FUNCTION_BLOCK FB_SboControl EXTENDS FB_AsyncServiceResultClass IMPLEMENTS I_AcsiDataAccessEventClass, I_AcsiDataAccessCompletionClass
VAR
	(* Interface pointer to controllable DO *)
	_ipCtrl					: I_AcsiCommonControllableDataClass;
	(* CDC type of the controllable DO *)
	_eType					: E_AcsiCDCType;
	(* Interface pointer to value of 'Beh' DO of parent LN *)
	_ipBehVal				: I_AcsiDATypeBeh;
	(* Interface pointer to DO containing stepsize information for BAC *)
	_ipStepSize				: I_AcsiDATypeAnalogueValue;
	
	(* State of control state machine *)
	_eControlState			: E_SboControlState;
	(* Interface pointer to association for the current control procedure *)
	_ipCurrentAA			: I_ScsmAssociationClass;
	(* IP address of the client for the current control procedure *)
	_stCurrrentIp			: ST_SockAddr;
	(* Timer to monitor 'sboTimeout' *)
	_fbSboTimer				: TON;
	
	(* Interface pointer to LastApplError request service *)
	_ipLastApplErrorReq		: I_AsyncServiceResultClass;
	(* State of LastApplError transmission *)
	_nLastApplErrorReqState	: BYTE;
	(* Interface pointer to CommandTermination request service *)
	_ipCmdTermReq			: I_AsyncServiceResultClass;
	(* State of CommandTermination transmission *)
	_nCmdTermReqState		: BYTE;
	
	(* Indicates whether this function block has been initialized *)
	bInit					: BOOL;
	(* Indicates whether the ControlState changed in the last cycle *)
	bNewState				: BOOL;
	(* Indicates whether a valid Oper_req was received *)
	bOperReq				: BOOL;
	(* Indicates whether a valid SelVal_req was received *)
	bSelValReq					: BOOL;
	(* Indicates whether a valid Cancel_req was received *)
	bCancelReq				: BOOL;
	(* Token for CompletionWaitEvent *)
	fbCompletion			: FB_AcsiServiceResultClass;
	(* Token for CompletionWaitEvent of SelVal_req *)
	fbSelValCompletion		: FB_AcsiServiceResultClass;
	(* Token for CompletionWaitEvent of Oper_req *)
	fbOperCompletion		: FB_AcsiServiceResultClass;
	(* Token for CompletionWaitEvent of Cancel_req *)
	fbCancelCompletion		: FB_AcsiServiceResultClass;
END_VAR

(*
	This method is called when Cancel_req is received.
	It shall check whether the Cancel request is valid and return FALSE as well as an error code if it is not.
*)
METHOD PROTECTED _CheckCancelReq : BOOL
VAR_INPUT
	(* Additional data access info *)
	ipDai			: I_AcsiDataAccessInfoClass;
END_VAR
VAR_OUTPUT
	(* Error code for negative response *)
	eError			: E_AcsiServiceError;
END_VAR
VAR
	(* Interface pointer to application association *)
	ipAA			: I_ScsmAssociationClass;
	(* Address of the client that sent the Cancel_req *)
	stRemoteAddr	: ST_SockAddr;
END_VAR
IF (_ipCtrl <> 0) AND_THEN (_ipCtrl.ipCancel <> 0) THEN
	ScsmAssociation_From_Dai(in:=ipDai, out=>ipAA);
	(* Don't allow control if 'ctlModel' is set to 'status-only' *)
	IF (_ipCtrl.ipCtlModel <> 0) AND_THEN (_ipCtrl.ipCtlModel.eValue = E_AcsiCtlModels.StatusOnly) THEN
		_SendLastApplError(ipAA:=ipAA,
			ipCtrlData:=_ipCtrl.ipCancel,
			eError:=E_AcsiApplError.NoError,
			ipOrigin:=_ipCtrl.ipCancel.ipOrigin,
			ipCtlNum:=_ipCtrl.ipCancel.ipCtlNum,
			eAddCause:=E_AcsiApplAddCause.Unknown);
		RETURN;
	
	(* Cancel is always allowed in state 'Unselected' *)
	ELSIF (_eControlState = E_SboControlState.Unselected) THEN
		_CheckCancelReq:=TRUE;
		RETURN;
	
	(* Cancel is only allowed by the same client that sent the last accepted SelVal_req *)
	ELSIF (RemoteAddress_From_ScsmAssociation(in:=ipAA, out=>stRemoteAddr)) AND_THEN (stRemoteAddr.sAddr <> _stCurrrentIp.sAddr) THEN
		_SendLastApplError(ipAA:=ipAA,
			ipCtrlData:=_ipCtrl.ipCancel,
			eError:=E_AcsiApplError.NoError,
			ipOrigin:=_ipCtrl.ipCancel.ipOrigin,
			ipCtlNum:=_ipCtrl.ipCancel.ipCtlNum,
			eAddCause:=E_AcsiApplAddCause.LockedByOtherClient);
		RETURN;
	
	(* Cancel is not allowed in state 'WaitForChange' *)
	ELSIF (_eControlState = E_SboControlState.WaitForChange) THEN
		_SendLastApplError(ipAA:=ipAA,
			ipCtrlData:=_ipCtrl.ipCancel,
			eError:=E_AcsiApplError.NoError,
			ipOrigin:=_ipCtrl.ipCancel.ipOrigin,
			ipCtlNum:=_ipCtrl.ipCancel.ipCtlNum,
			eAddCause:=E_AcsiApplAddCause.CommandAlreadyInExecution);
		RETURN;
	
	(* Cancel is valid *)
	ELSE
		_CheckCancelReq:=TRUE;
	END_IF
END_IF
END_METHOD

(*
	Checks if the value of 'ctlVal' is valid.
	Return value: TRUE => success, FALSE => failure
*)
METHOD PROTECTED _CheckCtlVal : BOOL
VAR_INPUT
	(* Value of 'ctlVal' DA *)
	uCtlVal			: U_AcsiCtlVal;
END_VAR
VAR_OUTPUT
	(* Error *)
	eError			: E_AcsiApplError;
	(* Application error code *)
	eAddCause		: E_AcsiApplAddCause;
END_VAR
IF (_ipCtrl = 0) OR_ELSE (_eType = E_AcsiCDCType.none) THEN
	RETURN;
END_IF

CASE _eType OF
	E_AcsiCDCType.SPC:
		IF (_ipCtrl.ipStVal_BOOLEAN = 0) THEN
			RETURN;
		END_IF
		IF (uCtlVal.SPC = _ipCtrl.ipStVal_BOOLEAN.bValue) THEN
			eError:=E_AcsiApplError.NoError;
			eAddCause:=E_AcsiApplAddCause.PositionReached;
		ELSE
			_CheckCtlVal:=TRUE;
		END_IF
	
	E_AcsiCDCType.DPC:
		IF (_ipCtrl.ipStVal_Dbpos = 0) THEN
			RETURN;
		END_IF
		IF ((SEL(uCtlVal.DPC, E_AcsiDbpos.Off, E_AcsiDbpos.On)) = _ipCtrl.ipStVal_Dbpos.eValue) THEN
			eError:=E_AcsiApplError.NoError;
			eAddCause:=E_AcsiApplAddCause.PositionReached;
		ELSE
			_CheckCtlVal:=TRUE;
		END_IF
	
	E_AcsiCDCType.INC:
		IF (_ipCtrl.ipStVal_INT32 = 0) THEN
			RETURN;
		END_IF
		IF (uCtlVal.INC = _ipCtrl.ipStVal_INT32.iValue) THEN
			eError:=E_AcsiApplError.NoError;
			eAddCause:=E_AcsiApplAddCause.PositionReached;
		ELSE
			_CheckCtlVal:=TRUE;
		END_IF
		
	E_AcsiCDCType.ENC:
		IF (_ipCtrl.ipStVal_ENUMERATED = 0) THEN
			RETURN;
		END_IF
		IF (uCtlVal.ENC.iAny = _ipCtrl.ipStVal_ENUMERATED.iAny) THEN
			eError:=E_AcsiApplError.NoError;
			eAddCause:=E_AcsiApplAddCause.PositionReached;
		ELSE
			_CheckCtlVal:=TRUE;
		END_IF
	
	E_AcsiCDCType.BSC:
		IF (_ipCtrl.ipValWTr = 0) THEN
			RETURN;
		END_IF
		CASE uCtlVal.BSC OF
			E_AcsiTcmd.Reserved:
				eError:=E_AcsiApplError.NoError;
				eAddCause:=E_AcsiApplAddCause.NotSupported;
			
			E_AcsiTcmd.Lower:
				IF (_ipCtrl.ipValWTr.iPosVal = -64) THEN
					eError:=E_AcsiApplError.NoError;
					eAddCause:=E_AcsiApplAddCause.StepLimit;
				ELSE
					_CheckCtlVal:=TRUE;
				END_IF
			
			E_AcsiTcmd.Higher:
				IF (_ipCtrl.ipValWTr.iPosVal = 63) THEN
					eError:=E_AcsiApplError.NoError;
					eAddCause:=E_AcsiApplAddCause.StepLimit;
				ELSE
					_CheckCtlVal:=TRUE;
				END_IF
			
			E_AcsiTcmd.Stop:
				_CheckCtlVal:=TRUE;
		END_CASE
	
	E_AcsiCDCType.ISC:
		IF (_ipCtrl.ipValWTr = 0) THEN
			RETURN;
		END_IF
		IF (uCtlVal.ISC < -64) OR_ELSE (uCtlVal.ISC > 63) THEN
			eError:=E_AcsiApplError.NoError;
			eAddCause:=E_AcsiApplAddCause.InconsistentParameters;
		ELSE
			_CheckCtlVal:=TRUE;
		END_IF
	
	E_AcsiCDCType.APC:
		IF (_ipCtrl.ipMxVal = 0) THEN
			RETURN;
		ELSE
			_CheckCtlVal:=TRUE;
		END_IF
	
	E_AcsiCDCType.BAC:
		IF (_ipCtrl.ipMxVal = 0) THEN
			RETURN;
		ELSE
			CASE uCtlVal.BAC OF
				E_AcsiTcmd.Reserved:
					eError:=E_AcsiApplError.NoError;
					eAddCause:=E_AcsiApplAddCause.NotSupported;
				
				ELSE
					_CheckCtlVal:=TRUE;
			END_CASE
		END_IF
END_CASE
END_METHOD

(*
	Checks if the values of two 'ctlVal' are equal.
	Return value: TRUE => equal, FALSE => unequal
*)
METHOD PROTECTED _CompareCtlVal : BOOL
VAR_INPUT
	(* Value of first 'ctlVal' *)
	uCtlVal1		: U_AcsiCtlVal;
	(* Value of second 'ctlVal' *)
	uCtlVal2		: U_AcsiCtlVal;
END_VAR
CASE _eType OF
	E_AcsiCDCType.SPC:
		_CompareCtlVal:=(uCtlVal1.SPC = uCtlVal2.SPC);
	
	E_AcsiCDCType.DPC:
		_CompareCtlVal:=(uCtlVal1.DPC = uCtlVal2.DPC);
	
	E_AcsiCDCType.INC:
		_CompareCtlVal:=(uCtlVal1.INC = uCtlVal2.INC);
	
	E_AcsiCDCType.ENC:
		_CompareCtlVal:=(uCtlVal1.ENC.iAny = uCtlVal2.ENC.iAny);
	
	E_AcsiCDCType.BSC:
		_CompareCtlVal:=(uCtlVal1.BSC = uCtlVal2.BSC);
	
	E_AcsiCDCType.ISC:
		_CompareCtlVal:=(uCtlVal1.ISC = uCtlVal2.ISC);
	
	E_AcsiCDCType.APC:
		_CompareCtlVal:=((uCtlVal1.APC.f = uCtlVal2.APC.f) AND_THEN (uCtlVal1.APC.i = uCtlVal2.APC.i));
	
	E_AcsiCDCType.BAC:
		_CompareCtlVal:=(uCtlVal1.BAC = uCtlVal2.BAC);
END_CASE
END_METHOD

(*
	This method performs the operative test.
	Since this test can take multiple PLC cycles, this method is called every cycle, until it returns TRUE.
*)
METHOD PROTECTED _DynamicTest : BOOL
VAR_OUTPUT
	(* Indicates whether the dynamic test was successful *)
	bDynamicTestOk	: BOOL;
	(* Error code for negative response *)
	eError			: E_AcsiServiceError;
END_VAR
bDynamicTestOk:=TRUE;
_DynamicTest:=TRUE;
END_METHOD

(* Initializes necessary local values *)
METHOD PROTECTED _Init
IF (_ipCtrl <> 0) THEN
	(* Set '_eType' according to CDC of the controllable data object *)
	IF (_ipCtrl.sClass = 'SPC') THEN
		_eType:=E_AcsiCDCType.SPC;
	ELSIF (_ipCtrl.sClass = 'DPC') THEN
		_eType:=E_AcsiCDCType.DPC;
	ELSIF (_ipCtrl.sClass = 'INC') THEN
		_eType:=E_AcsiCDCType.INC;
	ELSIF (_ipCtrl.sClass = 'ENC') THEN
		_eType:=E_AcsiCDCType.ENC;
	ELSIF (_ipCtrl.sClass = 'BSC') THEN
		_eType:=E_AcsiCDCType.BSC;
	ELSIF (_ipCtrl.sClass = 'ISC') THEN
		_eType:=E_AcsiCDCType.ISC;
	ELSIF (_ipCtrl.sClass = 'APC') THEN
		_eType:=E_AcsiCDCType.APC;
	ELSIF (_ipCtrl.sClass = 'BAC') THEN
		_eType:=E_AcsiCDCType.BAC;
	END_IF
END_IF
END_METHOD

(*
	This method performs the operative test.
	Since this test can take multiple PLC cycles, this method is called every cycle, until it returns TRUE.
*)
METHOD PROTECTED _OperativeTest : BOOL
VAR_OUTPUT
	(* Indicates whether the operative test was successful *)
	bOperativeTestOk	: BOOL;
	(* Error code for negative response *)
	eError				: E_AcsiServiceError;
END_VAR
VAR
	(* Error *)
	eApplError			: E_AcsiApplError;
	(* Application error code *)
	eApplAddCause		: E_AcsiApplAddCause;
END_VAR
IF (_ipCtrl <> 0) AND_THEN (_ipCtrl.ipOper <> 0) THEN
	(* Don't allow Oper_req if 'ctlModel' is set to 'status-only' *)
	IF (_ipCtrl.ipCtlModel <> 0) AND_THEN (_ipCtrl.ipCtlModel.eValue = E_AcsiCtlModels.StatusOnly) THEN
		_SendLastApplError(ipAA:=_ipCurrentAA,
			ipCtrlData:=_ipCtrl.ipOper,
			eError:=E_AcsiApplError.NoError,
			ipOrigin:=_ipCtrl.ipOper.ipOrigin,
			ipCtlNum:=_ipCtrl.ipOper.ipCtlNum,
			eAddCause:=E_AcsiApplAddCause.Unknown);
		eError:=E_AcsiServiceError.AccessViolation;
	
	(* Check if Oper_req is valid for current value of 'Beh' *)
	ELSIF (_ipBehVal <> 0) AND_THEN ((_ipBehVal.eValue = E_AcsiBeh.Off)
	OR_ELSE ((_ipCtrl.ipOper.ipTest <> 0) AND_THEN (_ipCtrl.ipOper.ipTest.bValue <> ((_ipBehVal.eValue = E_AcsiBeh.Test) OR_ELSE (_ipBehVal.eValue = E_AcsiBeh.TestBlocked))))) THEN
		_SendLastApplError(ipAA:=_ipCurrentAA,
			ipCtrlData:=_ipCtrl.ipOper,
			eError:=E_AcsiApplError.NoError,
			ipOrigin:=_ipCtrl.ipOper.ipOrigin,
			ipCtlNum:=_ipCtrl.ipOper.ipCtlNum,
			eAddCause:=E_AcsiApplAddCause.BlockedByMode);
		eError:=E_AcsiServiceError.AccessViolation;
	
	(* Check if 'ctlVal' is valid *)
	ELSIF (NOT _CheckCtlVal(uCtlVal:=_ipCtrl.ipOper.uCtlVal, eError=>eApplError, eAddCause=>eApplAddCause)) THEN
		_SendLastApplError(ipAA:=_ipCurrentAA,
			ipCtrlData:=_ipCtrl.ipOper,
			eError:=eApplError,
			ipOrigin:=_ipCtrl.ipOper.ipOrigin,
			ipCtlNum:=_ipCtrl.ipOper.ipCtlNum,
			eAddCause:=eApplAddCause);
		eError:=E_AcsiServiceError.AccessViolation;
	
	(* Oper_req is valid *)
	ELSE
		bOperativeTestOk:=TRUE;
	END_IF
END_IF
_OperativeTest:=TRUE;
END_METHOD

(* Resets all local values *)
METHOD PROTECTED _Reset
(* Reset local values *)
_ipCurrentAA:=0;
_stCurrrentIp.sAddr:='';
_stCurrrentIp.nPort:=0;
(* Reset timer *)
_fbSboTimer(IN:=FALSE);
END_METHOD

(* Resets all values of the 'Cancel' DA to their configured initial values. *)
METHOD PROTECTED _ResetCancelValues
VAR
	(* Interface pointer to 'Cancel' DA *)
	ipCancel		: I_AcsiDATypeCancel;
END_VAR
IF (_ipCtrl = 0) OR_ELSE ((ipCancel:=_ipCtrl.ipCancel) = 0) THEN
	RETURN;
END_IF

IF (ipCancel.ipCtlVal <> 0) THEN
	ipCancel.uCtlVal:=ipCancel.uCtlVal_Config;
END_IF
IF (ipCancel.ipOperTm <> 0) THEN
	ipCancel.ipOperTm.tValue:=ipCancel.ipOperTm.tConfig;
END_IF
IF (ipCancel.ipOrigin <> 0) THEN
	ipCancel.ipOrigin.stOrigin:=ipCancel.ipOrigin.stConfig;
END_IF
IF (ipCancel.ipCtlNum <> 0) THEN
	ipCancel.ipCtlNum.nValue:=ipCancel.ipCtlNum.nConfig;
END_IF
IF (ipCancel.ipT <> 0) THEN
	ipCancel.ipT.tValue:=ipCancel.ipT.tConfig;
END_IF
IF (ipCancel.ipTest <> 0) THEN
	ipCancel.ipTest.bValue:=ipCancel.ipTest.bConfig;
END_IF
END_METHOD

(* Resets all values of the 'Oper' DA to their configured initial values. *)
METHOD PROTECTED _ResetOperValues
VAR
	(* Interface pointer to 'Oper' DA *)
	ipOper			: I_AcsiDATypeOper;
END_VAR
IF (_ipCtrl = 0) OR_ELSE ((ipOper:=_ipCtrl.ipOper) = 0) THEN
	RETURN;
END_IF

IF (ipOper.ipCtlVal <> 0) THEN
	ipOper.uCtlVal:=ipOper.uCtlVal_Config;
END_IF
IF (ipOper.ipOperTm <> 0) THEN
	ipOper.ipOperTm.tValue:=ipOper.ipOperTm.tConfig;
END_IF
IF (ipOper.ipOrigin <> 0) THEN
	ipOper.ipOrigin.stOrigin:=ipOper.ipOrigin.stConfig;
END_IF
IF (ipOper.ipCtlNum <> 0) THEN
	ipOper.ipCtlNum.nValue:=ipOper.ipCtlNum.nConfig;
END_IF
IF (ipOper.ipT <> 0) THEN
	ipOper.ipT.tValue:=ipOper.ipT.tConfig;
END_IF
IF (ipOper.ipTest <> 0) THEN
	ipOper.ipTest.bValue:=ipOper.ipTest.bConfig;
END_IF
IF (ipOper.ipCheck <> 0) THEN
	ipOper.ipCheck.eValue:=ipOper.ipCheck.eConfig;
END_IF
END_METHOD

(* Resets all values of the 'SBOw' DA to their configured initial values. *)
METHOD PROTECTED _ResetSBOwValues
VAR
	(* Interface pointer to 'SBOw' DA *)
	ipSBOw			: I_AcsiDATypeSBOw;
END_VAR
IF (_ipCtrl = 0) OR_ELSE ((ipSBOw:=_ipCtrl.ipSBOw) = 0) THEN
	RETURN;
END_IF

IF (ipSBOw.ipCtlVal <> 0) THEN
	ipSBOw.uCtlVal:=ipSBOw.uCtlVal_Config;
END_IF
IF (ipSBOw.ipOperTm <> 0) THEN
	ipSBOw.ipOperTm.tValue:=ipSBOw.ipOperTm.tConfig;
END_IF
IF (ipSBOw.ipOrigin <> 0) THEN
	ipSBOw.ipOrigin.stOrigin:=ipSBOw.ipOrigin.stConfig;
END_IF
IF (ipSBOw.ipCtlNum <> 0) THEN
	ipSBOw.ipCtlNum.nValue:=ipSBOw.ipCtlNum.nConfig;
END_IF
IF (ipSBOw.ipT <> 0) THEN
	ipSBOw.ipT.tValue:=ipSBOw.ipT.tConfig;
END_IF
IF (ipSBOw.ipTest <> 0) THEN
	ipSBOw.ipTest.bValue:=ipSBOw.ipTest.bConfig;
END_IF
IF (ipSBOw.ipCheck <> 0) THEN
	ipSBOw.ipCheck.eValue:=ipSBOw.ipCheck.eConfig;
END_IF
END_METHOD

(* Sends a negative CommandTermination request *)
METHOD PROTECTED _SendCommandTerminationReqNeg : BOOL
VAR_INPUT
	(* Interface pointer to application association *)
	ipAA			: I_ScsmAssociationClass;
	(* Interface pointer to 'Oper', 'Cancel' or 'SBOw' control object, e.g. 'Relay1/XCBR1.CO.Pos.Oper', 'Relay1/CSWI1.CO.Pos.Cancel', 'Relay1/XCBR1.CO.Pos.SBOw' *)
	ipCtrlData		: I_AcsiCommonDataClass;
	(* Error *)
	eError			: E_AcsiApplError;
	(* Interface pointer to 'origin' attribute *)
	ipOrigin		: I_AcsiDATypeOriginator;
	(* Interface pointer to 'ctlNum' attribute *)
	ipCtlNum		: I_AcsiBAtypeINT8U;
	(* Application error code *)
	eAddCause		: E_AcsiApplAddCause;
END_VAR
VAR
	ipLastApplError	:I_AcsiDATypeLastApplError;
END_VAR
IF (ipAA <> 0)
AND_THEN (ipCtrlData <> 0)
AND_THEN (ipOrigin <> 0)
AND_THEN (ipCtlNum <> 0) THEN
	ipLastApplError:=ipAA.SetAdditionalCauseDiag(ipCtrlData:=ipCtrl,
		eError:=eError,
		stOrigin:=ipOrigin.stOrigin,
		nCtlNum:=ipCtlNum.nValue,
		eAddCause:=eAddCause);
	ipAA.CommandTerminationReq(ipCtrlData:=ipCtrlData,
		ipLastApplError:=ipLastApplError,
		ipResult=>_ipCmdTermReq);
	_nCmdTermReqState:=1;
END_IF
END_METHOD

(* Sends a positive CommandTermination request *)
METHOD PROTECTED _SendCommandTerminationReqPos : BOOL
VAR_INPUT
	(* Interface pointer to application association *)
	ipAA			: I_ScsmAssociationClass;
	(* Interface pointer to 'Oper', 'Cancel' or 'SBOw' control object, e.g. 'Relay1/XCBR1.CO.Pos.Oper', 'Relay1/CSWI1.CO.Pos.Cancel', 'Relay1/XCBR1.CO.Pos.SBOw' *)
	ipCtrlData		: I_AcsiCommonDataClass;
END_VAR
IF (ipAA <> 0)
AND_THEN (ipCtrlData <> 0) THEN
	_SendCommandTerminationReqPos:=ipAA.CommandTerminationReq(ipCtrlData:=ipCtrlData,
		ipLastApplError:=0,
		ipResult=>_ipCmdTermReq);
	_nCmdTermReqState:=1;
END_IF
END_METHOD

(* Sends a LastApplError request *)
METHOD PROTECTED _SendLastApplError : BOOL
VAR_INPUT
	(* Interface pointer to application association *)
	ipAA			: I_ScsmAssociationClass;
	(* Interface pointer to 'Oper', 'Cancel' or 'SBOw' control object *)
	ipCtrlData		: I_AcsiCommonDataClass;
	(* Error *)
	eError			: E_AcsiApplError;
	(* Interface pointer to 'origin' attribute *)
	ipOrigin		: I_AcsiDATypeOriginator;
	(* Interface pointer to 'ctlNum' attribute *)
	ipCtlNum		: I_AcsiBAtypeINT8U;
	(* Application error code *)
	eAddCause		: E_AcsiApplAddCause;
END_VAR
VAR
	(* Interface pointer to AdditionalCauseDiag object *)
	ipLastApplError	: I_AcsiDATypeLastApplError;
END_VAR
(* Get values from data and send LastApplError *)
IF (ipAA <> 0) AND_THEN (ipOrigin <> 0) AND_THEN (ipCtlNum <> 0) THEN
	ipLastApplError:=ipAA.SetAdditionalCauseDiag(ipCtrlData:=ipCtrlData,
		eError:=eError,
		stOrigin:=ipOrigin.stOrigin,
		nCtlNum:=ipCtlNum.nValue,
		eAddCause:=eAddCause);
		
	_SendLastApplError:=ipAA.LastApplErrorReq(ipLastApplError:=ipLastApplError, ipResult=>_ipLastApplErrorReq);
	SUPER^.SetBusy();
	_nLastApplErrorReqState:=1;
END_IF
END_METHOD

(*
	Sets the value of 'mxVal' to the value of 'ctlVal'.
	Return value: TRUE => success, FALSE => failure
*)
METHOD PROTECTED _SetApcValue : BOOL
VAR_INPUT
	(* Interface pointer to DA that will be written *)
	ipMxVal			: I_AcsiDATypeAnalogueValue;
	(* Value of 'ctlVal' DA *)
	uCtlVal			: U_AcsiCtlVal;
	(* Interface pointer to 'ctlVal' of type AnalogueValue *)
	ipCtlVal_AV		: I_AcsiDATypeAnalogueValue;
END_VAR
VAR
END_VAR
IF ((ipMxVal = 0) OR_ELSE ((ipMxVal.ipF = 0) AND_THEN (ipMxVal.ipI = 0)))
OR_ELSE ((ipCtlVal_AV = 0) OR_ELSE ((ipCtlVal_AV.ipF = 0) AND_THEN (ipCtlVal_AV.ipI = 0))) THEN
	RETURN;
END_IF

IF (ipMxVal.ipF <> 0) THEN
	IF (ipCtlVal_AV.ipF <> 0) THEN
		ipMxVal.fValue:=uCtlVal.APC.f;
	ELSE
		(* 'ctlVal.i' is present, but not 'ctlVal.f' -> convert and use value of 'ctlVal.i' *)
		ipMxVal.fValue:=DINT_TO_REAL(uCtlVal.APC.i);
	END_IF
END_IF
IF (ipMxVal.ipI <> 0) THEN
	IF (ipCtlVal_AV.ipI <> 0) THEN
		ipMxVal.iValue:=uCtlVal.APC.i;
	ELSE
		(* 'ctlVal.f' is present, but not 'ctlVal.i' -> convert and use value of 'ctlVal.f' *)
		ipMxVal.iValue:=REAL_TO_DINT(uCtlVal.APC.f);
	END_IF
END_IF
_SetApcValue:=TRUE;
END_METHOD

(*
	Increments or decrements the value of 'mxVal' according to the value of 'ctlVal' and 'stepSize'.
	If 'stepSize' is not specified, the value 1 is used.
	Return value: TRUE => success, FALSE => failure
*)
METHOD PROTECTED _SetBacValue : BOOL
VAR_INPUT
	(* Interface pointer to DA that will be written *)
	ipMxVal			: I_AcsiDATypeAnalogueValue;
	(* Value of 'ctlVal' DA *)
	uCtlVal			: U_AcsiCtlVal;
	(* Interface pointer to 'stepSize' DA (Optional) *)
	ipStepSize		: I_AcsiDATypeAnalogueValue;
END_VAR
VAR
	(* stepSize for 'f' *)
	fStepSize		: REAL:=1.0;
	(* stepSize for 'i' *)
	iStepSize		: DINT:=1;
END_VAR
IF (ipMxVal = 0) OR_ELSE ((ipMxVal.ipF = 0) AND_THEN (ipMxVal.ipI = 0)) THEN
	RETURN;
END_IF

IF (ipStepSize <> 0) AND_THEN (((ipStepSize.ipF <> 0) AND_THEN (ipStepSize.fValue <> 0.0)) OR_ELSE ((ipStepSize.ipI <> 0) AND_THEN (ipStepSize.iValue <> 0))) THEN
	IF (ipStepSize.ipF <> 0) THEN
		fStepSize:=ipStepSize.fValue;
	ELSE
		(* 'stepSize.i' is present, but not 'stepSize.f' -> convert and use value of 'stepSize.i' *)
		fStepSize:=DINT_TO_REAL(ipStepSize.iValue);
	END_IF
	IF (ipStepSize.ipI <> 0) THEN
		iStepSize:=ipStepSize.iValue;
	ELSE
		(* 'stepSize.f' is present, but not 'stepSize.i' -> convert and use value of 'stepSize.f' *)
		iStepSize:=REAL_TO_DINT(ipStepSize.fValue);
	END_IF
END_IF

CASE uCtlVal.BAC OF
	E_AcsiTcmd.Stop:
		_SetBacValue:=TRUE;
	
	E_AcsiTcmd.Lower:
		IF (ipMxVal.ipF <> 0) THEN
			ipMxVal.fValue:=ipMxVal.fValue - fStepSize;
		END_IF
		IF (ipMxVal.ipI <> 0) THEN
			ipMxVal.iValue:=ipMxVal.iValue - iStepSize;
		END_IF
		_SetBacValue:=TRUE;
	
	E_AcsiTcmd.Higher:
		IF (ipMxVal.ipF <> 0) THEN
			ipMxVal.fValue:=ipMxVal.fValue + fStepSize;
		END_IF
		IF (ipMxVal.ipI <> 0) THEN
			ipMxVal.iValue:=ipMxVal.iValue + iStepSize;
		END_IF
		_SetBacValue:=TRUE;
END_CASE
END_METHOD

(*
	Increments or decrements the value of 'valWTr' according to the value of 'ctlVal'.
	Return value: TRUE => success, FALSE => failure
*)
METHOD PROTECTED _SetBscValue : BOOL
VAR_INPUT
	(* Interface pointer to DA that will be written *)
	ipValWTr		: I_AcsiDATypeValWithTrans;
	(* Value of 'ctlVal' DA *)
	uCtlVal			: U_AcsiCtlVal;
END_VAR
VAR
END_VAR
IF (ipValWTr = 0) THEN
	RETURN;
END_IF

CASE uCtlVal.BSC OF
	E_AcsiTcmd.Stop:
		_SetBscValue:=TRUE;
	
	E_AcsiTcmd.Lower:
		ipValWTr.iPosVal:=ipValWTr.iPosVal - 1;
		_SetBscValue:=TRUE;
	
	E_AcsiTcmd.Higher:
		ipValWTr.iPosVal:=ipValWTr.iPosVal + 1;
		_SetBscValue:=TRUE;
END_CASE
END_METHOD

(*
	Sets the value of 'stVal' according to the value of 'ctlVal'.
	Return value: TRUE => success, FALSE => failure
*)
METHOD PROTECTED _SetDpcValue : BOOL
VAR_INPUT
	(* Interface pointer to DA that will be written *)
	ipStVal			: I_AcsiDATypeDbpos;
	(* Value of 'ctlVal' DA *)
	uCtlVal			: U_AcsiCtlVal;
END_VAR
VAR
END_VAR
IF (ipStVal = 0) THEN
	RETURN;
END_IF

ipStVal.eValue:=SEL(uCtlVal.DPC, E_AcsiDbpos.Off, E_AcsiDbpos.On);
_SetDpcValue:=TRUE;
END_METHOD

(*
	Sets the value of 'stVal' to the value of 'ctlVal'.
	Return value: TRUE => success, FALSE => failure
*)
METHOD PROTECTED _SetEncValue : BOOL
VAR_INPUT
	(* Interface pointer to DA that will be written *)
	ipStVal			: I_AcsiBATypeENUMERATED;
	(* Value of 'ctlVal' DA *)
	uCtlVal			: U_AcsiCtlVal;
END_VAR
VAR
END_VAR
IF (ipStVal = 0) THEN
	RETURN;
END_IF

ipStVal.iAny:=uCtlVal.ENC.iAny;
_SetEncValue:=TRUE;
END_METHOD

(*
	Sets the value of 'stVal' to the value of 'ctlVal'.
	Return value: TRUE => success, FALSE => failure
*)
METHOD PROTECTED _SetIncValue : BOOL
VAR_INPUT
	(* Interface pointer to DA that will be written *)
	ipStVal			: I_AcsiBATypeINT32;
	(* Value of 'ctlVal' DA *)
	uCtlVal			: U_AcsiCtlVal;
END_VAR
VAR
END_VAR
IF (ipStVal = 0) THEN
	RETURN;
END_IF

ipStVal.iValue:=uCtlVal.INC;
_SetIncValue:=TRUE;
END_METHOD

(*
	Sets the value of 'valWTr' to the value of 'ctlVal'.
	Return value: TRUE => success, FALSE => failure
*)
METHOD PROTECTED _SetIscValue : BOOL
VAR_INPUT
	(* Interface pointer to DA that will be written *)
	ipValWTr		: I_AcsiDATypeValWithTrans;
	(* Value of 'ctlVal' DA *)
	uCtlVal			: U_AcsiCtlVal;
END_VAR
VAR
END_VAR
IF (ipValWTr = 0) THEN
	RETURN;
END_IF

ipValWTr.iPosVal:=uCtlVal.ISC;
_SetIscValue:=TRUE;
END_METHOD

(*
	Sets the value of 'stVal' to the value of 'ctlVal'.
	Return value: TRUE => success, FALSE => failure
*)
METHOD PROTECTED _SetSpcValue : BOOL
VAR_INPUT
	(* Interface pointer to DA that will be written *)
	ipStVal			: I_AcsiBATypeBOOLEAN;
	(* Value of 'ctlVal' DA *)
	uCtlVal			: U_AcsiCtlVal;
END_VAR
VAR
END_VAR
IF (ipStVal = 0) THEN
	RETURN;
END_IF

ipStVal.bValue:=uCtlVal.SPC;
_SetSpcValue:=TRUE;
END_METHOD

(*
	Sets the value of the respective DA according to the value of 'Oper.ctlVal'.
	Return value: TRUE => success, FALSE => failure
*)
METHOD PROTECTED _SetValue : BOOL
VAR_INPUT
	(* Value of 'ctlVal' DA *)
	uCtlVal			: U_AcsiCtlVal;
	(* Interface pointer to 'ctlVal' of type AnalogueValue *)
	ipCtlVal_AV		: I_AcsiDATypeAnalogueValue;
END_VAR
IF (_ipCtrl = 0) THEN
	RETURN;
END_IF

CASE _eType OF
	E_AcsiCDCType.SPC:
		_SetValue:=_SetSpcValue(ipStVal:=_ipCtrl.ipStVal_BOOLEAN, uCtlVal:=uCtlVal);
	
	E_AcsiCDCType.DPC:
		_SetValue:=_SetDpcValue(ipStVal:=_ipCtrl.ipStVal_Dbpos, uCtlVal:=uCtlVal);
	
	E_AcsiCDCType.INC:
		_SetValue:=_SetIncValue(ipStVal:=_ipCtrl.ipStVal_INT32, uCtlVal:=uCtlVal);
	
	E_AcsiCDCType.ENC:
		_SetValue:=_SetEncValue(ipStVal:=_ipCtrl.ipStVal_ENUMERATED, uCtlVal:=uCtlVal);
	
	E_AcsiCDCType.BSC:
		_SetValue:=_SetBscValue(ipValWTr:=_ipCtrl.ipValWTr, uCtlVal:=uCtlVal);
	
	E_AcsiCDCType.ISC:
		_SetValue:=_SetIscValue(ipValWTr:=_ipCtrl.ipValWTr, uCtlVal:=uCtlVal);
	
	E_AcsiCDCType.APC:
		_SetValue:=_SetApcValue(ipMxVal:=_ipCtrl.ipMxVal, uCtlVal:=uCtlVal, ipCtlVal_AV:=ipCtlVal_AV);
	
	E_AcsiCDCType.BAC:
		_SetValue:=_SetBacValue(ipMxVal:=_ipCtrl.ipMxVal, uCtlVal:=uCtlVal, ipStepSize:=_ipStepSize);
END_CASE
END_METHOD

(*
	This method performs the test of the SelectWithValue operation.
	Since this test can take multiple PLC cycles, this method is called every cycle, until it returns TRUE.
*)
METHOD PROTECTED _Test : BOOL
VAR_OUTPUT
	(* Indicates whether the test was successful *)
	bTestOk				: BOOL;
	(* Error code for negative response *)
	eError				: E_AcsiServiceError;
END_VAR
VAR
	(* Error *)
	eApplError			: E_AcsiApplError;
	(* Application error code *)
	eApplAddCause		: E_AcsiApplAddCause;
END_VAR
IF (_ipCtrl <> 0) AND_THEN (_ipCtrl.ipSBOw <> 0) THEN
	(* Don't allow control if 'ctlModel' is set to 'status-only' *)
	IF (_ipCtrl.ipCtlModel <> 0) AND_THEN (_ipCtrl.ipCtlModel.eValue = E_AcsiCtlModels.StatusOnly) THEN
		_SendLastApplError(ipAA:=_ipCurrentAA,
			ipCtrlData:=_ipCtrl.ipSBOw,
			eError:=E_AcsiApplError.NoError,
			ipOrigin:=_ipCtrl.ipSBOw.ipOrigin,
			ipCtlNum:=_ipCtrl.ipSBOw.ipCtlNum,
			eAddCause:=E_AcsiApplAddCause.Unknown);
		eError:=E_AcsiServiceError.AccessViolation;
	
	(* Check if 'ctlVal' is valid *)
	ELSIF (NOT _CheckCtlVal(uCtlVal:=_ipCtrl.ipSBOw.uCtlVal, eError=>eApplError, eAddCause=>eApplAddCause)) THEN
		_SendLastApplError(ipAA:=_ipCurrentAA,
			ipCtrlData:=_ipCtrl.ipSBOw,
			eError:=eApplError,
			ipOrigin:=_ipCtrl.ipSBOw.ipOrigin,
			ipCtlNum:=_ipCtrl.ipSBOw.ipCtlNum,
			eAddCause:=eApplAddCause);
		eError:=E_AcsiServiceError.AccessViolation;
	
	(* SelVal_req is valid *)
	ELSE
		RemoteAddress_From_ScsmAssociation(in:=_ipCurrentAA, out=>_stCurrrentIp);
		bTestOk:=TRUE;
	END_IF
END_IF
_Test:=TRUE;
END_METHOD

(*
	Sets the value of 't' to the current time.
	Return value: TRUE => success, FALSE => failure
*)
METHOD PROTECTED _UpdateTimestampValue : BOOL
VAR_INPUT
	(* Interface pointer to application association *)
	ipAA			: I_ScsmAssociationClass;
END_VAR
VAR
	(* Current time *)
	tValue			: T_UtcTime;
END_VAR
IF (ipAA <> 0) AND_THEN (_ipCtrl <> 0) AND_THEN (_ipCtrl.ipT <> 0) THEN
	_UpdateTimestampValue:=ipAA.GetSystemTime(tT=>tValue);
	_ipCtrl.ipT.tValue:=tValue;
END_IF
END_METHOD

PROPERTY eType : E_AcsiCDCType
GET
eType:=_eType;
END_GET
SET
_eType:=eType;
END_SET
END_PROPERTY

METHOD Execute : BOOL
VAR
	(* Used to cache the return value of the last '_Test', '_OperativeTest' or '_DynamicTest' method call *)
	bTestOk	: BOOL;
	(* Used to cache the returned error of the last '_Test', '_OperativeTest' or '_DynamicTest' method call *)
	eError	: E_AcsiServiceError;
	
	(* Used to cache the current system time for 'tOpOk' *)
	tValue	: T_UtcTime;
END_VAR
IF (_ipCtrl <> 0) AND_THEN (_ipCtrl.ipOper <> 0) THEN
	(* Initialize function block in the first cycle *)
	IF NOT bInit THEN
		_Init();
		bInit:=TRUE;
	END_IF
	
	CASE _eControlState OF
		E_SboControlState.Unselected:
			(* Check if ControlState changed in the last cycle *)
			IF bNewState THEN
				bNewState:=FALSE;
				_Reset();
			END_IF
			(* Check if a valid Cancel_req was received *)
			IF bCancelReq THEN
				bCancelReq:=FALSE;
			END_IF
			(* Check if a valid SelVal_req was received *)
			IF bSelValReq THEN
				bSelValReq:=FALSE;
				(* Go to next ControlState *)
				_eControlState:=E_SboControlState.Select_PerformTest;
				bNewState:=TRUE;
			END_IF
		
		E_SboControlState.Select_PerformTest:
			(* Check if ControlState changed in the last cycle *)
			IF bNewState THEN
				bNewState:=FALSE;
			END_IF
			(* Trigger the test until it is finished *)
			IF _Test(bTestOk=>bTestOk, eError=>eError) THEN
				IF bTestOk THEN
					(* Go to next ControlState *)
					_eControlState:=E_SboControlState.WaitForSelection;
				ELSE
					fbSelValCompletion.SetCompleted();
					fbSelValCompletion.eServiceError:=eError;
					(* Go back to ControlState 'Unselected' *)
					_eControlState:=E_SboControlState.Unselected;
				END_IF
				bNewState:=TRUE;
			END_IF
		
		E_SboControlState.WaitForSelection:
			(* Check if ControlState changed in the last cycle *)
			IF bNewState THEN
				bNewState:=FALSE;
			END_IF
			(* Set 'stSeld' *)
			IF (_ipCtrl.ipStSeld <> 0) THEN
				_ipCtrl.ipStSeld.bValue:=TRUE;
			END_IF
			fbSelValCompletion.SetCompleted();
			(* Go to next ControlState *)
			_eControlState:=E_SboControlState.Ready;
			bNewState:=TRUE;
		
		E_SboControlState.Ready:
			(* Check if ControlState changed in the last cycle *)
			IF bNewState THEN
				bNewState:=FALSE;
				(* Start timer *)
				IF (_ipCtrl.ipSboTimeout <> 0) THEN
					_fbSboTimer(IN:=TRUE, PT:=DWORD_TO_TIME(_ipCtrl.ipSboTimeout.nValue));
				END_IF
			END_IF
			_fbSboTimer();
			(* Check if a valid Cancel_req was received, 'sboTimeout' was exceeded or the association was lost *)
			IF bCancelReq OR_ELSE _fbSboTimer.Q OR_ELSE ((_ipCurrentAA <> 0) AND_THEN (_ipCurrentAA.eState <> E_AsyncEnvironmentState.Established)) THEN
				bCancelReq:=FALSE;
				_fbSboTimer(IN:=FALSE);
				(* Go to next ControlState *)
				_eControlState:=E_SboControlState.EndSelection;
				bNewState:=TRUE;
			END_IF
			(* Check if a valid Oper_req was received *)
			IF bOperReq THEN
				bOperReq:=FALSE;
				(* Go to next ControlState *)
				_eControlState:=E_SboControlState.PerformTest;
				bNewState:=TRUE;
			END_IF
		
		E_SboControlState.PerformTest:
			(* Check if ControlState changed in the last cycle *)
			IF bNewState THEN
				bNewState:=FALSE;
				(* Set 'opRcvd' *)
				IF (_ipCtrl.ipOpRcvd <> 0) THEN
					_ipCtrl.ipOpRcvd.bValue:=TRUE;
				END_IF
			END_IF
			(* Check if a valid Cancel_req was received *)
			IF bCancelReq THEN
				bCancelReq:=FALSE;
				(* Send Oper_resp- *)
				_SendLastApplError(ipAA:=_ipCurrentAA,
					ipCtrlData:=_ipCtrl.ipOper,
					eError:=E_AcsiApplError.NoError,
					ipOrigin:=_ipCtrl.ipOper.ipOrigin,
					ipCtlNum:=_ipCtrl.ipOper.ipCtlNum,
					eAddCause:=E_AcsiApplAddCause.AbortionByCancel);
				fbOperCompletion.SetCompleted();
				fbOperCompletion.eServiceError:=E_AcsiServiceError.AccessViolation;
				(* Go to ControlState 'EndSelection' *)
				_eControlState:=E_SboControlState.EndSelection;
				bNewState:=TRUE;
			END_IF
			(* Trigger the operative test until it is finished *)
			IF _OperativeTest(bOperativeTestOk=>bTestOk, eError=>eError) THEN
				(* Reset 'opRcvd' *)
				IF (_ipCtrl.ipOpRcvd <> 0) THEN
					_ipCtrl.ipOpRcvd.bValue:=FALSE;
				END_IF
				IF bTestOk THEN
					(* Go to next ControlState *)
					_eControlState:=E_SboControlState.WaitForExecution;
				ELSE
					fbOperCompletion.SetCompleted();
					fbOperCompletion.eServiceError:=eError;
					(* Go to ControlState 'EndSelection' *)
					_eControlState:=E_SboControlState.EndSelection;
				END_IF
				bNewState:=TRUE;
			END_IF
		
		E_SboControlState.WaitForExecution:
			(* Check if ControlState changed in the last cycle *)
			IF bNewState THEN
				bNewState:=FALSE;
			END_IF
			(* Check if a Cancel_req was received *)
			IF bCancelReq THEN
				bCancelReq:=FALSE;
				(* Send Oper_resp- *)
				_SendLastApplError(ipAA:=_ipCurrentAA,
					ipCtrlData:=_ipCtrl.ipOper,
					eError:=E_AcsiApplError.NoError,
					ipOrigin:=_ipCtrl.ipOper.ipOrigin,
					ipCtlNum:=_ipCtrl.ipOper.ipCtlNum,
					eAddCause:=E_AcsiApplAddCause.AbortionByCancel);
				fbOperCompletion.SetCompleted();
				fbOperCompletion.eServiceError:=E_AcsiServiceError.AccessViolation;
				(* Go to ControlState 'EndSelection' *)
				_eControlState:=E_SboControlState.EndSelection;
				bNewState:=TRUE;
			END_IF
			(* Trigger the dynamic test until it is finished *)
			IF _DynamicTest(bDynamicTestOk=>bTestOk, eError=>eError) THEN
				fbOperCompletion.SetCompleted();
				IF bTestOk THEN
					(* Go to next ControlState *)
					IF (_ipBehVal <> 0) AND_THEN ((_ipBehVal.eValue = E_AcsiBeh.TestBlocked) OR_ELSE (_ipBehVal.eValue = E_AcsiBeh.OnBlocked)) THEN
						_eControlState:=E_SboControlState.MirrorBlockedCommand;
					ELSE
						_eControlState:=E_SboControlState.WaitForChange;
					END_IF
				ELSE
					fbOperCompletion.eServiceError:=eError;
					(* Go to ControlState 'EndSelection' *)
					_eControlState:=E_SboControlState.EndSelection;
				END_IF
				bNewState:=TRUE;
			END_IF
		
		E_SboControlState.WaitForChange:
			(* Check if ControlState changed in the last cycle *)
			IF bNewState THEN
				bNewState:=FALSE;
				(* Set 'opOk' *)
				IF (_ipCtrl.ipOpOk <> 0) THEN
					_ipCtrl.ipOpOk.bValue:=TRUE;
				END_IF
				(* Set 'tOpOk' *)
				IF (_ipCtrl.ipTOpOk <> 0) AND_THEN (_ipCurrentAA <> 0) AND_THEN (_ipCurrentAA.GetSystemTime(tT=>tValue)) THEN
					_ipCtrl.ipTOpOk.tValue:=tValue;
				END_IF
			END_IF
			(* Update value *)
			_SetValue(uCtlVal:=_ipCtrl.ipOper.uCtlVal, ipCtlVal_AV:=_ipCtrl.ipOper.ipCtlVal_AnalogueValue);
			(* Update Timestamp 't' *)
			_UpdateTimestampValue(ipAA:=_ipCurrentAA);
			
			(* Reset 'opOk' *)
			IF (_ipCtrl.ipOpOk <> 0) THEN
				_ipCtrl.ipOpOk.bValue:=FALSE;
			END_IF
			(* Send CmdTerm_req+ *)
			_SendCommandTerminationReqPos(ipAA:=_ipCurrentAA, ipCtrlData:=_ipCtrl.ipOper);
			(* Go to next ControlState *)
			IF (_ipCtrl.ipSboClass <> 0) AND_THEN (_ipCtrl.ipSboClass.eValue = E_AcsiSboClasses.OperateMany) THEN
				_eControlState:=E_SboControlState.Ready;
			ELSE
				_eControlState:=E_SboControlState.EndSelection;
			END_IF
			bNewState:=TRUE;
		
		E_SboControlState.MirrorBlockedCommand:
			(* Check if ControlState changed in the last cycle *)
			IF bNewState THEN
				bNewState:=FALSE;
				(* Set 'opOk' *)
				IF (_ipCtrl.ipOpOk <> 0) THEN
					_ipCtrl.ipOpOk.bValue:=TRUE;
				END_IF
				(* Set 'tOpOk' *)
				IF (_ipCtrl.ipTOpOk <> 0) AND_THEN (_ipCurrentAA <> 0) AND_THEN (_ipCurrentAA.GetSystemTime(tT=>tValue)) THEN
					_ipCtrl.ipTOpOk.tValue:=tValue;
				END_IF
			END_IF
			(* Reset 'opOk' *)
			IF (_ipCtrl.ipOpOk <> 0) THEN
				_ipCtrl.ipOpOk.bValue:=FALSE;
			END_IF
			(* Send CmdTerm_req- *)
			_SendCommandTerminationReqNeg(ipAA:=_ipCurrentAA,
				ipCtrlData:=_ipCtrl.ipOper,
				eError:=E_AcsiApplError.NoError,
				ipOrigin:=_ipCtrl.ipOper.ipOrigin,
				ipCtlNum:=_ipCtrl.ipOper.ipCtlNum,
				eAddCause:=E_AcsiApplAddCause.BlockedByMode);
			(* Go to next ControlState *)
			IF (_ipCtrl.ipSboClass <> 0) AND_THEN (_ipCtrl.ipSboClass.eValue = E_AcsiSboClasses.OperateMany) THEN
				_eControlState:=E_SboControlState.Ready;
			ELSE
				_eControlState:=E_SboControlState.EndSelection;
			END_IF
			bNewState:=TRUE;
		
		E_SboControlState.EndSelection:
			(* Check if ControlState changed in the last cycle *)
			IF bNewState THEN
				bNewState:=FALSE;
				(* Reset 'stSeld' *)
				IF (_ipCtrl.ipStSeld <> 0) THEN
					_ipCtrl.ipStSeld.bValue:=FALSE;
				END_IF
			END_IF
			(* Go to next ControlState *)
			_eControlState:=E_SboControlState.Unselected;
			bNewState:=TRUE;
	END_CASE
END_IF

(* Monitor transmission of LastApplError *)
CASE _nLastApplErrorReqState OF
	0:	;
	1:
		IF (_ipLastApplErrorReq <> 0) THEN
			Execute:=_ipLastApplErrorReq.Execute();
			IF NOT _ipLastApplErrorReq.IsBusy() THEN
				IF _ipLastApplErrorReq.IsCompleted() THEN
					SUPER^.SetCompleted();
				ELSE
					SUPER^.CopyFrom(ipSource:=_ipLastApplErrorReq);
				END_IF
				_nLastApplErrorReqState:=0;
			END_IF
		END_IF
END_CASE
(* Monitor transmission of CommandTermination *)
CASE _nCmdTermReqState OF
	0:	RETURN;
	1:
		IF (_ipCmdTermReq <> 0) THEN
			Execute:=_ipCmdTermReq.Execute();
			IF NOT _ipCmdTermReq.IsBusy() THEN
				IF _ipCmdTermReq.IsCompleted() THEN
					SUPER^.SetCompleted();
				ELSE
					SUPER^.CopyFrom(ipSource:=_ipLastApplErrorReq);
				END_IF
				_nCmdTermReqState:=0;
			END_IF
		END_IF
END_CASE
END_METHOD

PROPERTY ipBehVal : I_AcsiDATypeBeh
GET
ipBehVal:=_ipBehVal;
END_GET
SET
_ipBehVal:=ipBehVal;
END_SET
END_PROPERTY

PROPERTY ipCtrl : I_AcsiCommonControllableDataClass
GET
ipCtrl:=_ipCtrl;
END_GET
SET
IF (ipCtrl=0) THEN
	RETURN;
END_IF
_ipCtrl:=ipCtrl;
ipCtrl.ipEventSink:=THIS^;
END_SET
END_PROPERTY

PROPERTY ipStepSize : I_AcsiDATypeAnalogueValue
GET
ipStepSize:=_ipStepSize;
END_GET
SET
_ipStepSize:=ipStepSize;
END_SET
END_PROPERTY

METHOD OnAbort : BOOL
VAR_INPUT
	ipReason : I_ServiceErrorClass;
END_VAR
VAR_OUTPUT
	ipResult : I_AsyncServiceResultClass:=THIS^;
END_VAR
(* Forward Abort to LastApplError request service *)
IF (_ipLastApplErrorReq <> 0)AND_THEN (_ipLastApplErrorReq.IsBusy()) THEN
	_ipLastApplErrorReq.OnAbort(ipReason:=ipReason);
END_IF
(* Forward Abort to CommandTermination request service *)
IF (_ipCmdTermReq <> 0) AND_THEN (_ipCmdTermReq.IsBusy()) THEN
	_ipCmdTermReq.OnAbort(ipReason:=ipReason);
END_IF

SUPER^.SetCompleted();
fbCompletion.SetCompleted();
END_METHOD

(* TRUE => success, FALSE => failure *)
METHOD OnCompletionWaitEvent : BOOL
VAR_INPUT
	ipDai			: I_AcsiDataAccessInfoClass;
	ipData			: I_AcsiCommonDataClass;
	eFc				: E_AcsiFc;
END_VAR
VAR_OUTPUT
	ipResult		: I_AcsiServiceResultClass:=fbCompletion;
END_VAR
VAR
	eServiceError	: E_AcsiServiceError;
	(* Interface pointer to application association *)
	ipAA			: I_ScsmAssociationClass;
END_VAR
fbCompletion.SetCompleted();
IF (ipDai = 0) OR_ELSE (ipData = 0) THEN
	fbCompletion.eServiceError:=E_AcsiServiceError.AccessViolation;
	RETURN;
END_IF

(* Check if an Operate request is received *)
IF (ipDai.eService = E_AcsiServiceType.SetDataValues) THEN
	IF	(ipData.sObjectName = 'Oper') THEN
		fbOperCompletion.SetBusy();
		ipResult:=fbOperCompletion;
		bOperReq:=TRUE;
		OnCompletionWaitEvent:=TRUE;
	ELSIF (ipData.sObjectName = 'SBOw') THEN
		ScsmAssociation_From_Dai(in:=ipDai, out=>_ipCurrentAA);
		fbSelValCompletion.SetBusy();
		ipResult:=fbSelValCompletion;
		bSelValReq:=TRUE;
		OnCompletionWaitEvent:=TRUE;
	ELSIF (ipData.sObjectName = 'Cancel') THEN
		fbCancelCompletion.SetCompleted();
		ipResult:=fbCancelCompletion;
		IF _CheckCancelReq(ipDai:=ipDai, eError=>eServiceError) THEN
			bCancelReq:=TRUE;
		ELSE
			fbCancelCompletion.eServiceError:=eServiceError;
		END_IF
	END_IF
END_IF
END_METHOD

(* Implementation of user application data update event method. *)
METHOD OnGetVEvent
VAR_INPUT
	ipDai			: I_AcsiDataAccessInfoClass;(* Additional data access info *)
	ipData			: I_AcsiCommonDataClass;(* Interface pointer to data object *)
	eFc				: E_AcsiFc;(* Functional constraint *)
END_VAR
END_METHOD

(* Implementation of user application data update event method. *)
METHOD OnGetVPreEvent : E_AcsiServiceError
VAR_INPUT
	ipDai			: I_AcsiDataAccessInfoClass;(* Additional data access info *)
	ipData			: I_AcsiCommonDataClass;(* Interface pointer to data object *)
	eFc				: E_AcsiFc;(* Functional constraint *)
END_VAR
END_METHOD

(* Implementation of user application data update event method. *)
METHOD OnSetVEvent
VAR_INPUT
	ipDai			: I_AcsiDataAccessInfoClass;(* Additional data access info *)
	ipData			: I_AcsiCommonDataClass;(* Interface pointer to data object *)
	eFc				: E_AcsiFc;(* Functional constraint *)
END_VAR
END_METHOD

(* Implementation of user application data update event method. *)
METHOD OnSetVPreEvent : E_AcsiServiceError
VAR_INPUT
	ipDai			: I_AcsiDataAccessInfoClass;(* Additional data access info *)
	ipMemory		: I_AnyMemoryBuffer;(* Interface pointer to buffer containig new value data *)
	ipData			: I_AcsiCommonDataClass;(* Interface pointer to data object *)
	eFc				: E_AcsiFc;(* Functional constraint *)
END_VAR
VAR_OUTPUT
	ipLastApplError	: I_AcsiDATypeLastApplError;(* IF <> 0 => send LastApplError request *)
END_VAR
VAR
	(* Interface pointer to application association *)
	ipAA			: I_ScsmAssociationClass;
	(* If TRUE => Checking object is sub-data object itself *)
	bItself			: BOOL;
END_VAR
IF (eFc = E_AcsiFc.CO) AND_THEN (_ipCtrl <> 0) AND_THEN (ipDai <> 0) AND_THEN (ipDai.Write) AND_THEN (ipDai.ipAccessData <> 0) AND_THEN (ipData <> 0)
AND_THEN ScsmAssociation_From_Dai(in:=ipDai, out=>ipAA) THEN
	IF (_ipCtrl.ipOper <> 0) AND_THEN (_ipCtrl.ipOper.ipOrigin <> 0) AND_THEN (_ipCtrl.ipOper.ipCtlNum <> 0) THEN
		(* Check for invalid write attemps to prevent 'Oper' from being overwritten while a control request is being executed *)
		IF (ipDai.ipAccessData.sObjectName = 'Oper') THEN
			(* Only allow 'Oper' requests in state 'Ready' *)
			IF (_eControlState <> E_SboControlState.Ready) THEN
				ipLastApplError:=ipAA.SetAdditionalCauseDiag(ipCtrlData:=_ipCtrl.ipOper,
					eError:=E_AcsiApplError.NoError,
					stOrigin:=_ipCtrl.ipOper.ipOrigin.stOrigin,
					nCtlNum:=_ipCtrl.ipOper.ipCtlNum.nValue,
					eAddCause:=E_AcsiApplAddCause.CommandAlreadyInExecution);
				OnSetVPreEvent:=E_AcsiServiceError.AccessViolation;
				RETURN;
			END_IF
		ELSIF (_ipCtrl.ipOper.HasDataSubObject(ipData:=ipDai.ipAccessData, bItself=>bItself) AND_THEN (NOT bItself)) THEN
			(* Don't allow write access to subdata of 'Oper'*)
			ipLastApplError:=ipAA.SetAdditionalCauseDiag(ipCtrlData:=_ipCtrl.ipOper,
				eError:=E_AcsiApplError.NoError,
				stOrigin:=_ipCtrl.ipOper.ipOrigin.stOrigin,
				nCtlNum:=_ipCtrl.ipOper.ipCtlNum.nValue,
				eAddCause:=E_AcsiApplAddCause.NotSupported);
			OnSetVPreEvent:=E_AcsiServiceError.AccessViolation;
			RETURN;
		END_IF
	END_IF
	IF (_ipCtrl.ipSBOw <> 0) AND_THEN (_ipCtrl.ipSBOw.ipOrigin <> 0) AND_THEN (_ipCtrl.ipSBOw.ipCtlNum <> 0) THEN
		(* Check for invalid write attemps to prevent 'SBOw' from being overwritten while a control request is being executed *)
		IF (ipDai.ipAccessData.sObjectName = 'SBOw') THEN
			(* Only allow 'SelectWithValue' requests in state 'Unselected' *)
			IF (_eControlState <> E_SboControlState.Unselected) THEN
				ipLastApplError:=ipAA.SetAdditionalCauseDiag(ipCtrlData:=_ipCtrl.ipSBOw,
					eError:=E_AcsiApplError.NoError,
					stOrigin:=_ipCtrl.ipSBOw.ipOrigin.stOrigin,
					nCtlNum:=_ipCtrl.ipSBOw.ipCtlNum.nValue,
					eAddCause:=E_AcsiApplAddCause.CommandAlreadyInExecution);
				OnSetVPreEvent:=E_AcsiServiceError.AccessViolation;
				RETURN;
			ELSIF (_ipCtrl.ipSBOw.HasDataSubObject(ipData:=ipDai.ipAccessData, bItself=>bItself) AND_THEN (NOT bItself)) THEN
				(* Don't allow write access to subdata of 'SBOw'*)
				ipLastApplError:=ipAA.SetAdditionalCauseDiag(ipCtrlData:=_ipCtrl.ipSBOw,
					eError:=E_AcsiApplError.NoError,
					stOrigin:=_ipCtrl.ipSBOw.ipOrigin.stOrigin,
					nCtlNum:=_ipCtrl.ipSBOw.ipCtlNum.nValue,
					eAddCause:=E_AcsiApplAddCause.NotSupported);
				OnSetVPreEvent:=E_AcsiServiceError.AccessViolation;
				RETURN;
			END_IF
		END_IF
	END_IF
	IF (_ipCtrl.ipCancel <> 0) AND_THEN (_ipCtrl.ipCancel.ipOrigin <> 0) AND_THEN (_ipCtrl.ipCancel.ipCtlNum <> 0) THEN
		IF (ipDai.ipAccessData.sObjectName <> 'Cancel') AND_THEN (_ipCtrl.ipCancel.HasDataSubObject(ipData:=ipDai.ipAccessData)) THEN
			(* Don't allow write access to subdata of 'Cancel'*)
			ipLastApplError:=ipAA.SetAdditionalCauseDiag(ipCtrlData:=_ipCtrl.ipCancel,
				eError:=E_AcsiApplError.NoError,
				stOrigin:=_ipCtrl.ipCancel.ipOrigin.stOrigin,
				nCtlNum:=_ipCtrl.ipCancel.ipCtlNum.nValue,
				eAddCause:=E_AcsiApplAddCause.NotSupported);
			OnSetVPreEvent:=E_AcsiServiceError.AccessViolation;
			RETURN;
		END_IF
	END_IF
END_IF
END_METHOD

END_FUNCTION_BLOCK
